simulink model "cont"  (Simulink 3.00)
settings: Solver=ode45  StartTime=0.0  StopTime=10.0  RelTol=1e-3
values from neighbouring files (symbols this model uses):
  A = [a11 a12 0 -g;a21 a22 1 0;a31 a31 a33 0;0 1 0 0]    [EXP7_3.M]    (also in EXP6_10.M = [0 1 0;0 -1.799 6.953;0 0.939 -1.660]; EXP6_8.M; EXP6_9.m; EXP7_1.M = [0 1 0 0;0 0 -mb*g/(1-mb) 0;0 0 0 1;0 0 m2_bar*g/(1-mb) 0])
  B = [b1;b2;b3;0]    [EXP7_3.M]    (also in EXP6_10.M = [0 0;-28.97 -6.453;-0.174 -0.230]; EXP6_8.M; EXP6_9.m; EXP7_1.M = [0;1/((m+M)*(1-mb));0;-m2_bar/((m+M)*(1-mb))])
  K = acker(A,B,Pc)    [EXP7_3.M]    (also in EXP6_10.M = Q*inv(V); EXP6_8.M = acker(A,B,P); EXP6_9.m = acker(A_bar,B_bar,P); Exp7_4.m = [0.922 -6.5955 -2.35 -8.977])
libraries: simulink3 x3

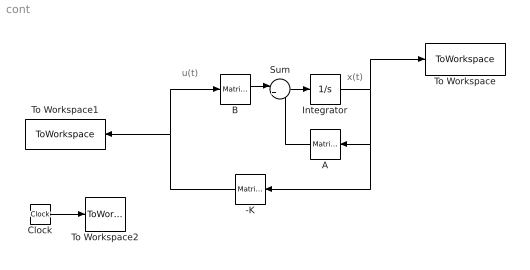
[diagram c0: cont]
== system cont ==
  note: x(t)
  note: u(t)
  -K : simulink3/Math/Matrix Gain  Orientation=left  K=-K
  A : simulink3/Math/Matrix Gain  Orientation=left  K=A
  B : simulink3/Math/Matrix Gain  K=B
  Clock : Clock
  Integrator : Integrator  ExternalReset=none  InitialConditionSource=internal  InitialCondition=[0.2 .1 -0.5 .5]  LimitOutput=off  UpperSaturationLimit=inf  LowerSaturationLimit=-inf  ShowSaturationPort=off  ShowStatePort=off  AbsoluteTolerance=auto
  Sum : Sum  Inputs=|++  SaturateOnIntegerOverflow=on
  To Workspace : ToWorkspace  VariableName=cont_states  SampleTime=-1  SaveFormat=Matrix
  To Workspace1 : ToWorkspace  VariableName=cont_control  SampleTime=-1  SaveFormat=Matrix
  To Workspace2 : ToWorkspace  VariableName=time1  SampleTime=-1  SaveFormat=Matrix
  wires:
  B/1 -> Sum/1
  Sum/1 -> Integrator/1
  Integrator/1 -> To Workspace/1, A/1, -K/1
  A/1 -> Sum/2
  Clock/1 -> To Workspace2/1
  -K/1 -> B/1, To Workspace1/1
